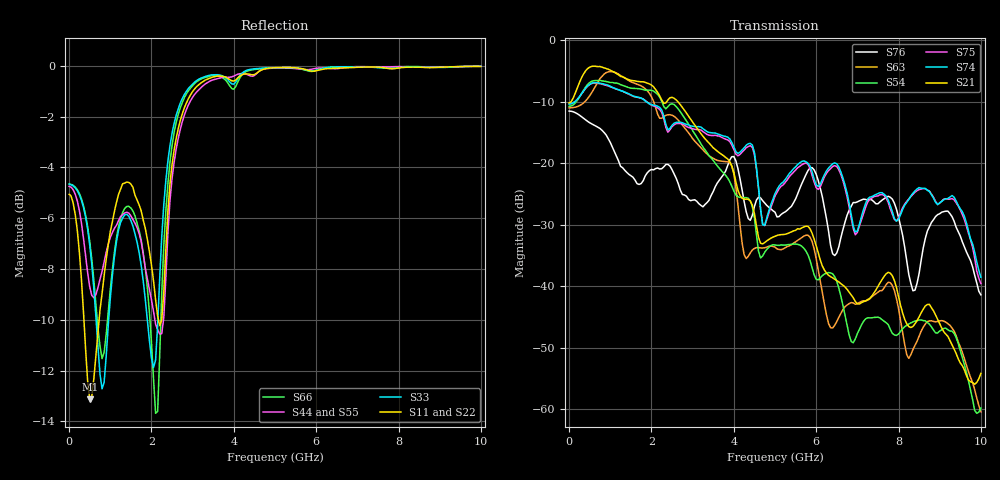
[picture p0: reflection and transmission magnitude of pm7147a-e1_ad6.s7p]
# GHz S DB R 50
! S-Parameters data
! Freq  dbS11  angS11  dbS12  angS12  dbS13  angS13  dbS14  angS14
!  dbS15  angS15  dbS16  angS16  dbS17  angS17  dbS21  angS21
!  dbS22  angS22  dbS23  angS23  dbS24  angS24  dbS25  angS25
!  dbS26  angS26  dbS27  angS27  dbS31  angS31  dbS32  angS32
!  dbS33  angS33  dbS34  angS34  dbS35  angS35  dbS36  angS36
!  dbS37  angS37  dbS41  angS41  dbS42  angS42  dbS43  angS43
!  dbS44  angS44  dbS45  angS45  dbS46  angS46  dbS47  angS47
!  dbS51  angS51  dbS52  angS52  dbS53  angS53  dbS54  angS54
!  dbS55  angS55  dbS56  angS56  dbS57  angS57  dbS61  angS61
!  dbS62  angS62  dbS63  angS63  dbS64  angS64  dbS65  angS65
!  dbS66  angS66  dbS67  angS67  dbS71  angS71  dbS72  angS72
!  dbS73  angS73  dbS74  angS74  dbS75  angS75  dbS76  angS76
!  dbS77  angS77
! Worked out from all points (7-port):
!   279 points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, 1 Hz to 10 GHz, reference 50 ohm
!   strongest paths, dB at 1 Hz, 7.943 MHz, 3.05 GHz, 6.55 GHz, 10 GHz:
!     S21: -10.1, -10.1, -13.7, -39.3, -54.1
!     S74: -10.3, -10.3, -14.0, -20.6, -38.5
!     S75: -10.3, -10.3, -14.4, -21.0, -39.5
!     S54: -10.7, -10.7, -15.2, -40.3, -59.8
!     S63: -11.0, -11.0, -16.4, -45.0, -60.4
!     S76: -11.5, -11.5, -25.9, -33.6, -41.4
!   lowest |S11| = -13.1 dB at 500 MHz (marker M1), VSWR 1.57, Z = 32 + j1.32 ohm
!   |S11| at or under -10 dB: 359.7 MHz to 727.2 MHz (367.5 MHz wide, 67.6 % of centre); 2.17 GHz to 2.251 GHz (80.72 MHz wide, 3.65 % of centre)
